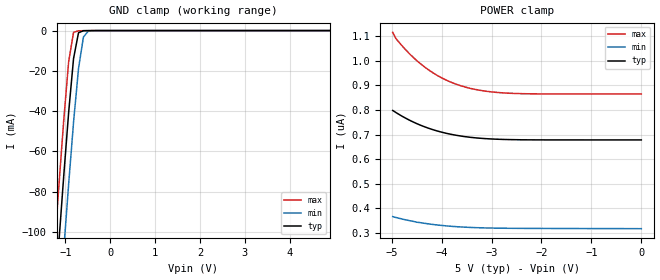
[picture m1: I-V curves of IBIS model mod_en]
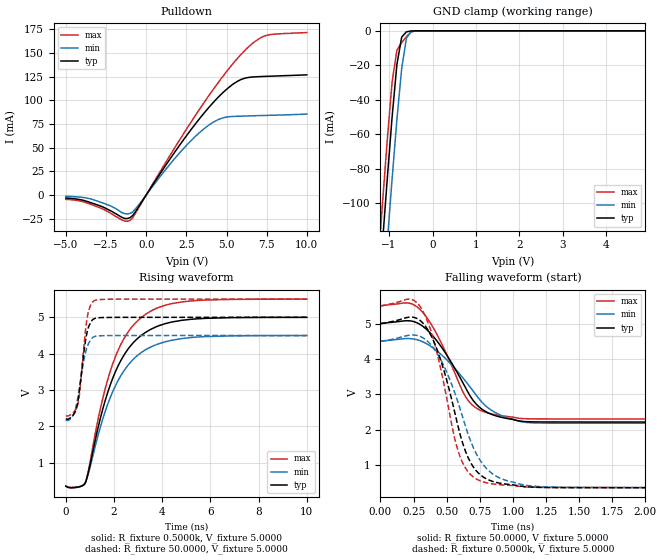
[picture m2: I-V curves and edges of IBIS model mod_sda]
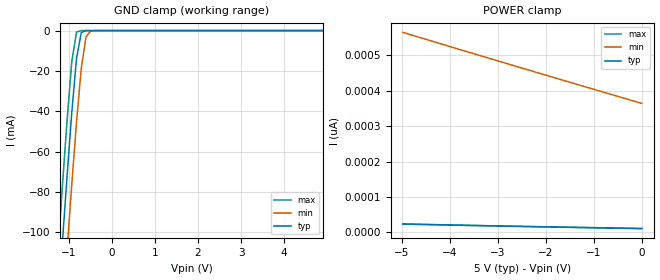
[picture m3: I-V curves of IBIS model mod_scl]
| IBIS (I/O, Buffer, Information, Specification) Model, officially
| electronic behavioral standard for Buffer structures of digital pins.
[IBIS ver]  4.0
[File name] m24c32_g6_tssop8.ibs
[File Rev]  1.0
[Date]   30 April 2015
[Source]   CAD & Design Services (Catania) - STMicroelectronics
[Notes]
   (Note1)  This IBIS model includes the TSSOP8 package data
   (Note2)  This IBIS model has some Notes about the non-monotonicity
   of the I-V curves, but they are not indicative of problems
   inside the model;
[Copyright] (c) 2015 STMicroelectronics
|   Component M24C32
[Component] M24C32
[Manufacturer] STMicroelectronics
[Package]
| variable  typ   min   max
R_pkg   0.0   0.0   0.0
L_pkg   0.0H   0.0H   0.0H
C_pkg   0.0F   0.0F   0.0F
[Pin]  signal_name   model_name   R_pin   L_pin   C_pin
1   E0   mod_en   NA   NA   NA
2   E1   mod_en   NA   NA   NA
3   E2   mod_en   NA   NA   NA
4   VSS   GND   NA   NA   NA
5   SDA   mod_sda   NA   NA   NA
6   SCL   mod_scl   NA   NA   NA
7   WCN   mod_wcn   NA   NA   NA
8   VCC   POWER   NA   NA   NA
[Package Model]  182696_TSSOP8
[Define Package Model]  182696_TSSOP8
[Manufacturer]  STMicroelectronics
[OEM]  STMicroelectronics
[Description]  8 pin TSSOP package
[Number Of Pins]  8
[Pin Numbers]
|Pin Num   Terminal Name
1   | net1
2   | net2
3   | net3
4   | net4_GND
5   | net5
6   | net6
7   | net7
8   | net8_VDD
[Model Data]
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[End Model Data]
[End Package Model]
| Models and submodels in the file (4): mod_en (Input), mod_sda (I/O_open_drain), mod_scl (Input), mod_wcn (Input)
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|   Model mod_en
[Model]   mod_en
Model_type Input
Vinl   =   1.500V
Vinh   =   3.500V
C_comp   2.119pF   2.023pF   2.323pF
[Temperature Range]   25.0000   0.1250k   -40.0000
[Voltage Range]   5.0000V   4.5000V   5.5000V
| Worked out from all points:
|   GND clamp passes 1 mA (typ) near -0.70 V on its own axis
[GND_clamp]
|Voltage   I(typ)   I(min)   I(max)
-5V       -1.381A    -1.415A    -1.356A
-1.26V    -140.4mA   -177.6mA   -112.3mA
-1.15V    -105.9mA   -143.1mA   -77.85mA
-1.04V    -72.4mA    -109.2mA   -44.81mA
-930mV    -40.73mA   -76.34mA   -15.55mA
-820mV    -13.84mA   -45.44mA   -867.4uA
-710mV    -1.105mA   -18.88mA   -97.48uA
-600mV    -55.62uA   -3.201mA   -59.79uA
-490mV    -14.19uA   -211.3uA   -30.28uA
4.9V      3.327uA    1.881uA    5.49uA
[POWER_clamp]
|Voltage   I(typ)   I(min)   I(max)
-4.98V    798.1nA    365.7nA    1.116uA
-4.92V    790.2nA    362.4nA    1.092uA
-4.74V    768.7nA    353.5nA    1.049uA
-4.5V     744.6nA    343nA      1.001uA
-4.32V    729.9nA    337.8nA    971.8nA
-4.08V    714nA      331.5nA    939.8nA
-3.9V     704.7nA    327.9nA    920.9nA
-3.72V    697.4nA    325nA      905.8nA
-3.48V    690.1nA    322.2nA    890.7nA
-3.06V    682.6nA    319.4nA    875nA
-2.58V    679.2nA    318.1nA    867.6nA
0V        678nA      316.7nA    865.1nA
|   Model mod_sda
[Model]   mod_sda
Model_type I/O_open_drain
Polarity   Inverting
Vinl   =   1.500V
Vinh   =   3.500V
Vmeas  =   2.500V
Cref   =   10pF
Rref   =   1k
Vref   =   5.000V
C_comp   2.925pF   2.667pF   3.207pF
[Temperature Range]   25.0000   0.1250k   -40.0000
[Voltage Range]   5.0000V   4.5000V   5.5000V
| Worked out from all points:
|   slope of the pulldown table from 0 to 0.75 V, typ, clamps not added: 38.4 ohm
|   GND clamp passes 1 mA (typ) near -0.62 V on its own axis
|   rising waveform, R_fixture 0.5000k, V_fixture 5.0000: 20-80 % time 1.41ns typ, 1.45ns min, 1.36ns max; typ from 0.354 V to 5 V
|   rising waveform, R_fixture 50.0000, V_fixture 5.0000: 20-80 % time 316ps typ, 365ps min, 282ps max; typ from 2.21 V to 5 V
|   falling waveform, R_fixture 50.0000, V_fixture 5.0000: 20-80 % time 272ps typ, 319ps min, 239ps max; typ from 5 V to 2.21 V
|   falling waveform, R_fixture 0.5000k, V_fixture 5.0000: 20-80 % time 208ps typ, 248ps min, 182ps max; typ from 5 V to 0.354 V
[Pulldown]
|Voltage   I(typ)   I(min)   I(max)
-5V       -3.214mA   -1.302mA   -4.574mA
-3.4V     -8.342mA   -4.36mA    -10.09mA
-1.48V    -23.85mA   -18.88mA   -26.56mA
-1V       -23.84mA   -19.3mA    -26.73mA
-520mV    -13.76mA   -11.59mA   -14.94mA
1.72V     43.83mA    37.38mA    48.3mA
3V        73.61mA    60.85mA    82.31mA
4.28V     99.55mA    77.79mA    113.9mA
5.24V     114.8mA    82.7mA     135.3mA
6.2V      123.5mA    83.38mA    153.5mA
7.32V     125.1mA    83.93mA    167.5mA
10V       126.8mA    85.45mA    171.4mA
[GND_clamp]
|Voltage   I(typ)   I(min)   I(max)
-5V       -1.535A    -1.568A    -1.514A
-1.26V    -160.6mA   -197.8mA   -137.7mA
-1.15V    -122.4mA   -159.6mA   -99.49mA
-1.04V    -85.2mA    -122.1mA   -62.66mA
-930mV    -49.9mA    -85.72mA   -29.63mA
-820mV    -19.54mA   -51.48mA   -11.22mA
-710mV    -3.664mA   -21.94mA   -6.819mA
-600mV    -560.4uA   -4.178mA   -3.354mA
-490mV    -78.82uA   -439.2uA   -616.8uA
-380mV    -6.109uA   -68.66uA   -6.344uA
4.9V      215.6pA    1.666nA    210.2pA
[Ramp]
| variable   typ   min   max
dV/dt_r  1.6710/0.3569n   1.3913/0.4118n   1.9194/0.3309n
dV/dt_f  1.6710/0.2971n   1.3913/0.3395n   1.9194/0.2634n
R_load = 50.0000
[Rising Waveform]
R_fixture= 0.5000k
V_fixture= 5.0000   | New T=105C (min)
V_fixture_min= 4.5000
V_fixture_max= 5.5000
|time   V(typ)   V(min)   V(max)
0s        353.7mV    361.8mV    359.2mV
460ps     326.6mV    324.7mV    337.4mV
800ps     438.5mV    444.7mV    435.9mV
1.47ns    2.324V     2.07V      2.599V
1.93ns    3.298V     2.934V     3.691V
2.49ns    4.042V     3.605V     4.503V
3.19ns    4.532V     4.059V     5.025V
4.13ns    4.827V     4.328V     5.334V
5.2ns     4.946V     4.444V     5.451V
10ns      5V         4.499V     5.5V
[Rising Waveform]
R_fixture= 50.0000
V_fixture= 5.0000   | New T=105 (min)
V_fixture_min= 4.5000
V_fixture_max= 5.5000
|time   V(typ)   V(min)   V(max)
0s        2.215V     2.181V     2.301V
320ps     2.329V     2.334V     2.389V
440ps     2.495V     2.597V     2.509V
500ps     2.682V     2.816V     2.624V
580ps     3.076V     3.15V      2.982V
760ps     4.1V       3.86V      4.288V
880ps     4.586V     4.179V     4.974V
980ps     4.794V     4.328V     5.253V
1.18ns    4.962V     4.468V     5.457V
10ns      5V         4.5V       5.5V
[Falling Waveform]
R_fixture= 50.0000
V_fixture= 5.0000   | New T=105 (min)
V_fixture_min= 4.5000
V_fixture_max= 5.5000
|time   V(typ)   V(min)   V(max)
0s        5V         4.5V       5.5V
200ps     5.081V     4.577V     5.586V
280ps     5.016V     4.54V      5.464V
360ps     4.794V     4.405V     5.118V
460ps     4.339V     4.121V     4.452V
620ps     3.343V     3.476V     3.088V
680ps     2.936V     3.191V     2.747V
840ps     2.431V     2.543V     2.445V
1.06ns    2.24V      2.228V     2.317V
10ns      2.215V     2.181V     2.301V
[Falling Waveform]
R_fixture= 0.5000k
V_fixture= 5.0000   | New T=105 (min)
V_fixture_min= 4.5000
V_fixture_max= 5.5000
|time   V(typ)   V(min)   V(max)
0s        5V         4.5V       5.5V
220ps     5.183V     4.673V     5.692V
300ps     5.089V     4.638V     5.484V
360ps     4.814V     4.486V     5.022V
440ps     4.138V     4.085V     3.974V
600ps     1.885V     2.606V     1.247V
700ps     951.5mV    1.505V     663.5mV
840ps     544.9mV    768.2mV    469.6mV
1.38ns    359.3mV    370.9mV    365.3mV
10ns      353.7mV    361.8mV    359.2mV
|   Model mod_scl
[Model]   mod_scl
Model_type Input
Vinl   =   1.500V
Vinh   =   3.500V
C_comp   2.119pF   2.023pF   2.323pF
[Temperature Range]   25.0000   0.1250k   -40.0000
[Voltage Range]   5.0000V   4.5000V   5.5000V
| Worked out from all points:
|   GND clamp passes 1 mA (typ) near -0.71 V on its own axis
[GND_clamp]
|Voltage   I(typ)   I(min)   I(max)
-5V       -1.38A     -1.414A    -1.355A
-1.26V    -140.2mA   -177.3mA   -112mA
-1.15V    -105.7mA   -142.8mA   -77.62mA
-1.04V    -72.25mA   -109mA     -44.62mA
-930mV    -40.6mA    -76.19mA   -15.4mA
-820mV    -13.75mA   -45.33mA   -741.8uA
-710mV    -1.045mA   -18.8mA    -5.45uA
-600mV    -23.09uA   -3.148mA   -36.27nA
-490mV    -459.2nA   -183.2uA   -242.2pA
4.9V      10.56pA    379.5pA    10.13pA
[POWER_clamp]
|Voltage   I(typ)   I(min)   I(max)
-4.98V    24.27pA    563.8pA    23.46pA
-3.96V    21.17pA    522.2pA    20.77pA
-2.64V    17.45pA    468.9pA    17.5pA
0V        10.79pA    363.7pA    11.44pA
